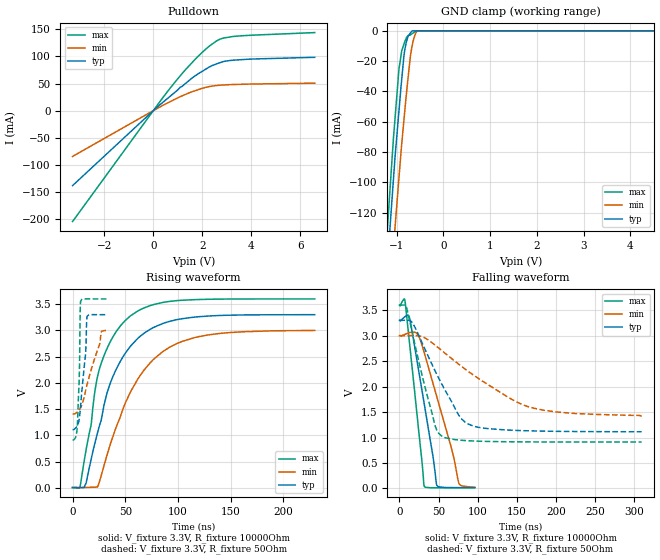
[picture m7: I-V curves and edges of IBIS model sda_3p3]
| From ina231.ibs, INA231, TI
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|   sda_3p3 Model
[Model]   sda_3p3
Model_type   I/O_open_drain
Polarity   Non-Inverting
Vinl = 0.4
Vinh = 1.4
Vmeas = 1.65
Vref = 3.3
Cref = 2pF
Rref = 10000
|   typ   min   max
|   (nom PVT)   (fast PVT)   (slow PVT)
|C_comp from frequency sweep method (F=100KHz)
|C_comp   2.585e-10   2.237e-10   2.895e-10
|ON state : BUFFER OUTPUT TURNED LOW
|C_comp   2.585e-10   2.237e-10   2.895e-10
|OFF state: BUFFER IN HIGH IMPEDANCE
|C_comp   2.386e-12   1.967e-12   2.887e-12
|C_comp from LC tank measurement(L=1nH)
|Resonant Frequency(Hz)   5.580e+09   5.710e+09   5.200e+09
C_comp   8.143e-13   7.777e-13   9.377e-13
|ON state : BUFFER OUTPUT TURNED LOW
|Resonant Frequency(Hz)   5.580e+09   5.710e+09   5.200e+09
|C_comp   8.143e-13   7.777e-13   9.377e-13
|OFF state: BUFFER IN HIGH IMPEDANCE
|Resonant Frequency(Hz)   4.900e+09   5.620e+09   4.490e+09
|C_comp   1.056e-12   8.028e-13   1.258e-12
| Where nom  PVT is Nominal Process, 3.3V, 27C
|   Fast PVT is Strong Process,  3.6V, -40C
|   Slow PVT is Weak Process,   3V, 125C
[Voltage Range]   3.3   3   3.6
|Ambient Temperature   25   150   -65
|Junction Temperature
[Temperature Range]   27   125   -40
[Pullup Reference]   3.3   3   3.6
[Pulldown Reference]   0   0   0
[Power Clamp Reference]   3.3   3   3.6
[GND Clamp Reference]   0   0   0
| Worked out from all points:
|   slope of the pulldown table from 0 to 0.495 V, typ, clamps not added: 25.6 ohm
|   GND clamp passes 1 mA (typ) near -0.70 V on its own axis
|   falling waveform, V_fixture 3.3V, R_fixture 10000Ohm: 20-80 % time 21.4ns typ, 32.6ns min, 14.7ns max; typ from 3.3 V to 0.014 V
|   rising waveform, V_fixture 3.3V, R_fixture 10000Ohm: 20-80 % time 33.8ns typ, 42.1ns min, 25.6ns max; typ from 0.008 V to 3.3 V
|   falling waveform, V_fixture 3.3V, R_fixture 50Ohm: 20-80 % time 42.9ns typ, 89.4ns min, 25.8ns max; typ from 3.3 V to 1.11 V
|   rising waveform, V_fixture 3.3V, R_fixture 50Ohm: 20-80 % time 5.35ns typ, 13.7ns min, 1.96ns max; typ from 1.11 V to 3.3 V
[Pulldown]
|   Voltage   I(typ)   I(min)   I(max)
-3.3V     -138.3mA   -84.45mA   -204.6mA
161.7mV   6.785mA    4.049mA    9.955mA
584.4mV   22.67mA    14.26mA    35.45mA
1.112V    43.77mA    25.93mA    64.88mA
1.29V     49.18mA    29.52mA    74.26mA
1.713V    64.28mA    36.84mA    94.82mA
2.291V    80.53mA    44.44mA    119.1mA
2.73V     88.55mA    46.98mA    131.9mA
3.259V    93.08mA    48.19mA    136.8mA
6.6V      98.43mA    50.73mA    144mA
[GND Clamp]
|   Voltage   I(typ)   I(min)   I(max)
-3.3V     -1.114A    -1.098A    -1.171A
-1.31V    -202mA     -242.1mA   -185.2mA
-1.18V    -145.7mA   -188.1mA   -121.6mA
-1.086V   -105.3mA   -149.4mA   -78.5mA
-1.033V   -82.48mA   -128.6mA   -56.9mA
-949.2mV  -52.11mA   -96.26mA   -24.86mA
-891.6mV  -31.8mA    -74.54mA   -13.05mA
-825mV    -12.24mA   -52.13mA   -7.054mA
-702mV    -1.217mA   -15.65mA   -2.606mA
-663.3mV  0A         -9.024mA   -1.739mA
-561mV    0A         -32.16uA   -180.3uA
6.6V      0A         0A         0A
[POWER Clamp]
|   Voltage   I(typ)   I(min)   I(max)
-3.3V     0A         0A         0A
0V        0A         0A         0A
6.6V      0A         0A         0A
[Ramp]
R_load = 10000
|   typ   min   max
dV/dt_r   1.97533/3.3778e-08   1.79298/4.20431e-08   2.15656/2.56148e-08
dV/dt_f   1.97216/2.14494e-08   1.79298/3.27894e-08   2.15322/1.47121e-08
[Falling Waveform]
V_fixture = 3.3V
V_fixture_min = 3V
V_fixture_max = 3.6V
R_fixture = 10000Ohm
|   Time   V(typ)   V(min)   V(max)
0s        3.3V       3V         3.6V
6ns       3.359V     3.019V     3.722V
7.4ns     3.375V     3.028V     3.648V
13.6ns    3.303V     3.063V     2.752V
23.8ns    2.384V     3.015V     1.253V
31.8ns    1.652V     2.661V     40.88mV
48.2ns    51.6mV     1.776V     12.94mV
68.2ns    16.33mV    685.4mV    11.96mV
75.8ns    15.46mV    110.7mV    11.8mV
96.2ns    14.33mV    26.2mV     11.55mV
[Rising Waveform]
V_fixture = 3.3V
V_fixture_min = 3V
V_fixture_max = 3.6V
R_fixture = 10000Ohm
|   Time   V(typ)   V(min)   V(max)
0s        7.784mV    11.69mV    5.725mV
7ns       5.863mV    10.43mV    9.195mV
12.8ns    90.51mV    11.42mV    724.1mV
17.6ns    544mV      13.32mV    1.198V
23.6ns    1.043V     18.56mV    2.113V
36.2ns    2.017V     855.6mV    2.801V
55.4ns    2.709V     1.844V     3.283V
76.2ns    3.05V      2.437V     3.489V
104ns     3.224V     2.791V     3.575V
229.8ns   3.3V       3V         3.6V
[Falling Waveform]
V_fixture = 3.3V
V_fixture_min = 3V
V_fixture_max = 3.6V
R_fixture = 50Ohm
|   Time   V(typ)   V(min)   V(max)
0s        3.3V       3V         3.6V
9ns       3.302V     3.001V     3.554V
18.8ns    3.194V     3.001V     2.893V
45.6ns    2.307V     2.813V     1.235V
55.8ns    2V         2.686V     1.013V
79.8ns    1.358V     2.392V     945.2mV
98.8ns    1.207V     2.181V     928.7mV
149.4ns   1.139V     1.7V       915mV
172.2ns   1.129V     1.574V     913.1mV
309.6ns   1.112V     1.418V     911.5mV
[Rising Waveform]
V_fixture = 3.3V
V_fixture_min = 3V
V_fixture_max = 3.6V
R_fixture = 50Ohm
|   Time   V(typ)   V(min)   V(max)
0s        1.112V     1.411V     911.7mV
4.4ns     1.181V     1.444V     1.133V
6.4ns     1.325V     1.487V     2.126V
7.2ns     1.465V     1.514V     3.344V
7.6ns     1.552V     1.529V     3.551V
12.4ns    2.574V     1.859V     3.601V
13.8ns    3.264V     1.971V     3.6V
25.8ns    3.3V       2.747V     3.6V
27.4ns    3.3V       2.979V     3.6V
32.98ns   3.3V       3V         3.6V
